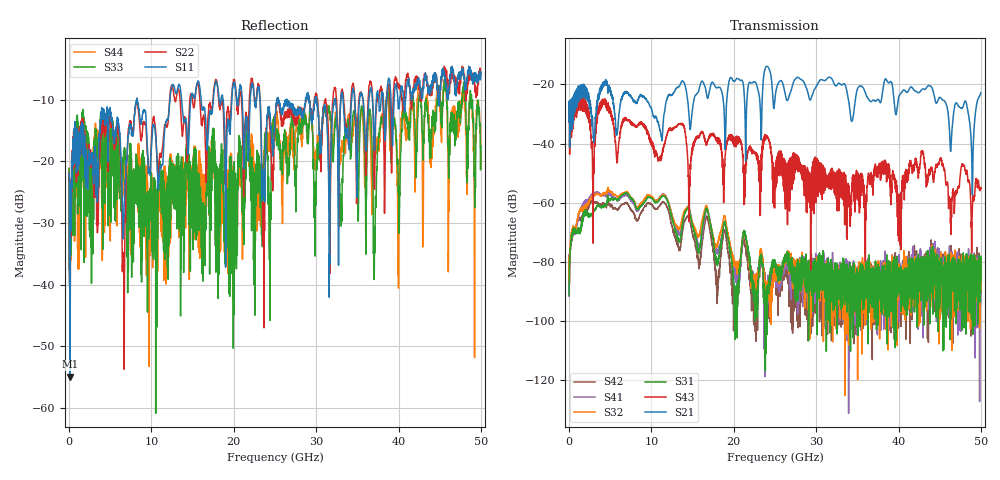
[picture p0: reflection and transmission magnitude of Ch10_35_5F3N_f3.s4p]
!Agilent Technologies,N5247A,US51170199,A.09.90.13
!Agilent N5247A: A.09.90.13
!Date: Wednesday, December 16, 2015 12:42:04
!Correction: S11(Full 4 Port(1,2,3,4))
!S12(Full 4 Port(1,2,3,4))
!S13(Full 4 Port(1,2,3,4))
!S14(Full 4 Port(1,2,3,4))
!S21(Full 4 Port(1,2,3,4))
!S22(Full 4 Port(1,2,3,4))
!S23(Full 4 Port(1,2,3,4))
!S24(Full 4 Port(1,2,3,4))
!S31(Full 4 Port(1,2,3,4))
!S32(Full 4 Port(1,2,3,4))
!S33(Full 4 Port(1,2,3,4))
!S34(Full 4 Port(1,2,3,4))
!S41(Full 4 Port(1,2,3,4))
!S42(Full 4 Port(1,2,3,4))
!S43(Full 4 Port(1,2,3,4))
!S44(Full 4 Port(1,2,3,4))
!S4P File: Measurements: <S11,S12,S13,S14>,
!<S21,S22,S23,S24>,
!<S31,S32,S33,S34>,
!<S41,S42,S43,S44>:
# Hz S  dB  R 50
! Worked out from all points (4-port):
!   3201 points, 10 MHz to 50 GHz, reference 50 ohm
!   strongest paths, dB at 10 MHz, 12.51 GHz, 25 GHz, 37.5 GHz, 50 GHz:
!     S21: -32.5, -23.4, -24.6, -25.0, -22.8
!     S43: -32.7, -34.9, -48.1, -48.5, -54.9
!     S31: -91.2, -65.3, -80.5, -84.9, -86.5
!     S32: -78.6, -64.5, -83.8, -87.3, -79.8
!     S41: -80.9, -63.8, -84.6, -88.2, -85.2
!     S42: -77.6, -67.8, -85.6, -90.0, -90.6
!   lowest |S11| = -55.0 dB at 135 MHz (marker M1), VSWR 1.00, Z = 50 + j0.172 ohm
!   |S11| at or under -10 dB: start of sweep to 8.23 GHz; 8.278 GHz to 12.26 GHz (3.977 GHz wide, 38.7 % of centre); 26.47 GHz to 28.71 GHz (2.24 GHz wide, 8.12 % of centre)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
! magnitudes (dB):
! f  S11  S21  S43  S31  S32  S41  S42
! 10 MHz  -22.0  -32.5  -32.7  -91.2  -78.6  -80.9  -77.6
! 135 MHz  -55.0  -32.8  -33.9  -76.2  -74.0  -74.2  -77.8
! 6.884 GHz  -22.3  -22.9  -31.9  -56.6  -56.2  -57.3  -60.0
! 12.49 GHz  -7.8  -23.6  -35.0  -65.3  -64.3  -64.2  -67.9
! 43.77 GHz  -8.4  -20.4  -50.5  -85.4  -93.5  -87.0  -85.2
! 48.94 GHz  -6.2  -51.9  -65.0  -83.9  -84.8  -83.6  -98.5
! 50 GHz  -5.6  -22.8  -54.9  -86.5  -79.8  -85.2  -90.6
